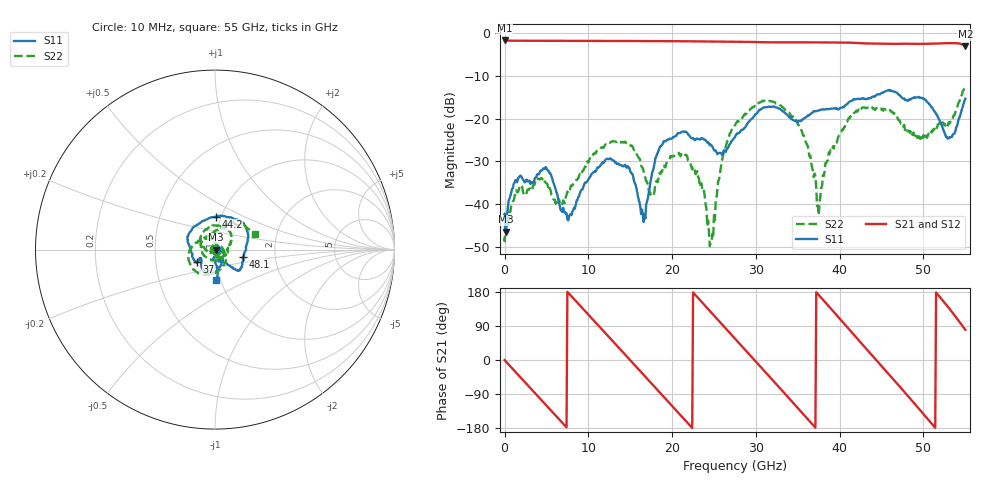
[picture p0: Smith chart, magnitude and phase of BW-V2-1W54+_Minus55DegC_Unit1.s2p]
!Mini-Circuits Laboratory
!S-Parameters
!Type: Fixed Attenuator
!Model: BW-V2-1W54+
!Run / Lot / Date Code: YE0105 / QN2150331 / 2150
!Fixture: N/A, Pressing Arm: N/A
!Network Analyzer: Keysight P9375A;  Serial number: 76634
!Date: 1/25/2022 at 8:22:18 AM
!S/N: Unit# 2 (U1 -55°C)
!Tested with: 2 PORT CALIBRATION USING eCAL. DE-EMBEDDED 1.85MM F/F ADAPTER ON PORT 1. TEMP AT -55°C.
!Remark: UNITS TESTED IN 50 OHM SYSTEM, WITHOUT Z-CONVERSION, PORT EXTENSION OFF.
# Hz  S  dB  R  50
!Frequency  S11 dB  S11 Deg  S21 dB  S21 Deg  S12 dB  S12 Deg  S22 dB  S22 Deg
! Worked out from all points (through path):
!   559 points, 10 MHz to 55 GHz, reference 50 ohm
!   highest |S21| = -1.66 dB at 10 MHz (marker M1); lowest = -3.0 dB at 55 GHz (marker M2)
!   group delay of S21, straight-line fit = 68.1 ps
!   lowest |S11| = -46.5 dB at 200 MHz (marker M3), VSWR 1.01, Z = 50.5 - j0.0583 ohm
!   |S11| at or under -10 dB: start of sweep to end of sweep
!   |S22| runs from -49.9 to -12.4 dB; largest |S21 - S12| = 0.0013
!   S11 on the Smith chart (normalised r, x): 10 MHz: 1.01, +0.01; 37 GHz: 0.81, -0.11; 44.2 GHz: 0.94, +0.36; 48.1 GHz: 1.37, -0.11; 55 GHz: 0.95, -0.34
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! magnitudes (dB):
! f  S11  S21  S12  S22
! 10 MHz  -43.4  -1.7  -1.7  -48.0
! 200 MHz  -46.5  -1.7  -1.7  -46.7
! 1.8 GHz  -33.5  -1.7  -1.7  -35.9
! 5.1 GHz  -32.0  -1.7  -1.7  -35.3
! 7.7 GHz  -43.0  -1.8  -1.8  -36.8
! 9.2 GHz  -36.7  -1.8  -1.8  -32.8
! 12.8 GHz  -29.6  -1.8  -1.8  -25.3
! 16.6 GHz  -44.2  -1.8  -1.8  -32.4
! 18.4 GHz  -27.3  -1.8  -1.8  -33.7
! 21.8 GHz  -23.3  -1.9  -1.9  -28.8
! 24.7 GHz  -26.3  -1.9  -1.9  -48.9
! 27.6 GHz  -23.8  -1.9  -1.9  -21.1
! 32.9 GHz  -17.8  -2.1  -2.1  -16.9
! 36.7 GHz  -18.6  -2.1  -2.1  -31.4
! 37 GHz  -18.2  -2.1  -2.1  -32.9
! 37.5 GHz  -18.1  -2.1  -2.1  -42.6
! 40.9 GHz  -16.6  -2.2  -2.2  -20.7
! 44.2 GHz  -14.8  -2.4  -2.4  -17.9
! 45.9 GHz  -13.3  -2.5  -2.5  -17.7
! 48.1 GHz  -15.8  -2.4  -2.4  -23.0
! 53 GHz  -24.6  -2.3  -2.3  -20.9
! 55 GHz  -15.3  -3.0  -3.0  -12.4
